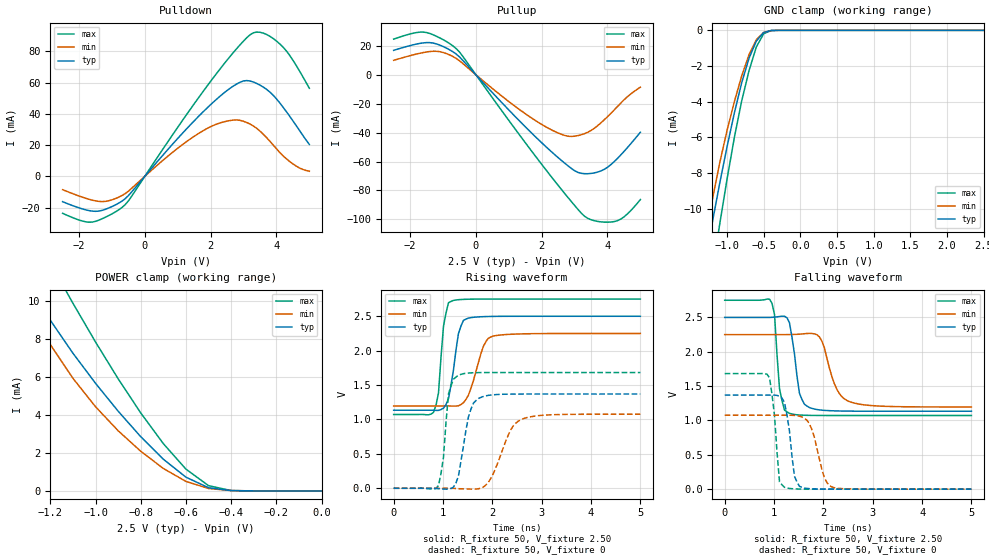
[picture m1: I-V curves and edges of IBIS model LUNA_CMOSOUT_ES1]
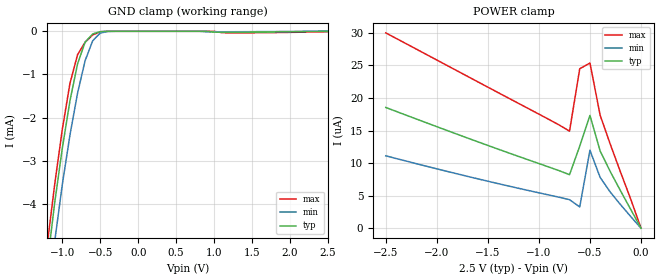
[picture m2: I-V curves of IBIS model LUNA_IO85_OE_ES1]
[IBIS Ver]   3.2
[Comment Char]   |_char
[File name]   sg-9101cx_25v_a.ibs
[File Rev]   1.0
[Date]   2018/09/14 17:35:48
[Source]
[Notes]
[Disclaimer]
This information is for modeling purposes only, and is not guaranteed.
Property of SEIKO EPSON Corp.,
unauthorized reproduction and/or distribution is strictly prohibited.
[Copyright]
Copyright 2018, SEIKO EPSON Corp.
[Component]   SG-9101CA
Si_location Pin
Timing_location Pin
[Manufacturer]   SEIKO EPSON Corp.
| 7050 PKG
| 7050 PKG
[Package]
R_pkg   224m   NA   NA
L_pkg   5.5n   NA   NA
C_pkg   0.144p   NA   NA
[Pin] signal_name   model_name
1   OE   LUNA_IO85_OE_ES1
2   VSS   GND
3   OUT   LUNA_CMOSOUT_ES1
4   VDD   POWER
[Component]   SG-9101CB
Si_location Pin
Timing_location Pin
[Manufacturer]   SEIKO EPSON Corp.
| 5032 PKG
| 5032 PKG
[Package]
R_pkg   200m   NA   NA
L_pkg   2.16n   NA   NA
C_pkg   1.23p   NA   NA
[Pin] signal_name   model_name
1   OE   LUNA_IO85_OE_ES1
2   VSS   GND
3   OUT   LUNA_CMOSOUT_ES1
4   VDD   POWER
[Component]   SG-9101CE
Si_location Pin
Timing_location Pin
[Manufacturer]   SEIKO EPSON Corp.
| 3225 PKG
| 3225 PKG
[Package]
R_pkg   177m   NA   NA
L_pkg   4.5n   NA   NA
C_pkg   0.64p   NA   NA
[Pin] signal_name   model_name
1   OE   LUNA_IO85_OE_ES1
2   VSS   GND
3   OUT   LUNA_CMOSOUT_ES1
4   VDD   POWER
[Component]   SG-9101CG
Si_location Pin
Timing_location Pin
[Manufacturer]   SEIKO EPSON Corp.
| 2520 PKG
| 2520 PKG
[Package]
R_pkg   238m   NA   NA
L_pkg   2.1n   NA   NA
C_pkg   0.38p   NA   NA
[Pin] signal_name   model_name
1   OE   LUNA_IO85_OE_ES1
2   VSS   GND
3   OUT   LUNA_CMOSOUT_ES1
4   VDD   POWER
| Models and submodels in the file (2): LUNA_CMOSOUT_ES1 (3-state), LUNA_IO85_OE_ES1 (Input)
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[Model]   LUNA_CMOSOUT_ES1
Model_type 3-state
Enable Active-High
Polarity Non-Inverting
Vmeas=1.25
C_comp   2.5p   2.0p   3.0p
[Temperature Range] 25   105   -40
[Voltage Range]   2.50   2.25   2.75
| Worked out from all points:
|   slope of the pulldown table from 0 to 0.375 V, typ, clamps not added: 40.3 ohm
|   slope of the pullup table from 0 to 0.375 V, typ, clamps not added: 40.5 ohm
|   GND clamp passes 1 mA (typ) near -0.64 V on its own axis
|   POWER clamp passes 1 mA (typ) near -0.63 V on its own axis
|   falling waveform, R_fixture 50, V_fixture 2.50: 20-80 % time 153ps typ, 284ps min, 106ps max; typ from 2.5 V to 1.13 V
|   falling waveform, R_fixture 50, V_fixture 0: 20-80 % time 142ps typ, 230ps min, 120ps max; typ from 1.37 V to 0 V
|   rising waveform, R_fixture 50, V_fixture 2.50: 20-80 % time 170ps typ, 265ps min, 115ps max; typ from 1.13 V to 2.5 V
|   rising waveform, R_fixture 50, V_fixture 0: 20-80 % time 207ps typ, 362ps min, 123ps max; typ from 0 V to 1.37 V
[Pullup]
-2.5V     16.88mA    9.98mA     24.65mA
-1.5V     22.23mA    15.75mA    29.19mA
-1.1V     20.51mA    15.96mA    25.51mA
-600mV    14.33mA    11.31mA    18.1mA
1.9V      -44.85mA   -32.97mA   -58.98mA
2.7V      -61.14mA   -41.98mA   -82.12mA
3.1V      -67.51mA   -42.09mA   -93.03mA
3.5V      -68.25mA   -38.54mA   -100.3mA
3.9V      -65.45mA   -31.2mA    -101.9mA
4.2V      -60.17mA   -24.44mA   -101.6mA
4.5V      -53.1mA    -17.42mA   -98.33mA
5V        -39.74mA   -8.599mA   -86.32mA
[Pulldown]
-2.5V     -16.25mA   -8.571mA   -23.68mA
-1.6V     -22.29mA   -15.27mA   -29.31mA
-1.1V     -20.31mA   -15.69mA   -25.16mA
-600mV    -14.4mA    -11.1mA    -18.2mA
900mV     21.89mA    16.28mA    28.28mA
1.9V      43.85mA    30.66mA    57.95mA
2.8V      59.13mA    36.05mA    81.88mA
3.3V      60.3mA     32.16mA    91.82mA
3.7V      55.62mA    24.74mA    90.75mA
4.2V      44.25mA    13.13mA    82.67mA
4.6V      32.45mA    6.521mA    70.93mA
5V        20.38mA    3.216mA    56.31mA
[GND Clamp]
-2.5V     -55.19mA   -49.46mA   -64.23mA
-1.3V     -13.11mA   -11.85mA   -16.24mA
-1.2V     -10.77mA   -9.503mA   -13.52mA
-1.1V     -8.591mA   -7.44mA    -10.88mA
-1V       -6.541mA   -5.623mA   -8.358mA
-900mV    -4.635mA   -4.001mA   -6.009mA
-800mV    -2.939mA   -2.563mA   -3.961mA
-700mV    -1.565mA   -1.365mA   -2.263mA
-600mV    -601.2uA   -521.6uA   -925.2uA
-500mV    -121.4uA   -116.4uA   -188.8uA
-300mV    -500.8nA   -1.29uA    -313.5nA
2.5V      140pA      621.1nA    98.8pA
[POWER Clamp]
-2.5V     46.99mA    40.94mA    56.3mA
-1.4V     13.2mA     11.93mA    16.56mA
-1.3V     10.93mA    9.714mA    14.21mA
-1.2V     8.97mA     7.69mA     11.99mA
-1.1V     7.236mA    5.92mA     9.861mA
-1V       5.655mA    4.424mA    7.824mA
-900mV    4.191mA    3.162mA    5.894mA
-700mV    1.665mA    1.179mA    2.483mA
-600mV    721.7uA    498.7uA    1.143mA
-500mV    167.2uA    126.9uA    275.1uA
-400mV    16.41uA    18.75uA    19.76uA
0V        140pA      780.7pA    121.2pA
[Falling Waveform]
R_fixture=50
V_fixture=2.50
V_fixture_min=2.25
V_fixture_max=2.75
0s        2.5V       2.25V      2.75V
959.6ps   2.502V     2.25V      2.704V
1.01ns    2.504V     2.25V      2.539V
1.111ns   2.513V     2.25V      1.46V
1.313ns   2.422V     2.251V     1.103V
1.515ns   1.395V     2.256V     1.079V
1.717ns   1.188V     2.268V     1.074V
1.97ns    1.15V      2.156V     1.073V
2.525ns   1.136V     1.275V     1.072V
5ns       1.134V     1.196V     1.072V
[Falling Waveform]
R_fixture=50
V_fixture=0
V_fixture_min=0
V_fixture_max=0
0s        1.37V      1.076V     1.682V
909.1ps   1.37V      1.076V     1.62V
1.01ns    1.369V     1.076V     1.067V
1.111ns   1.354V     1.076V     106.5mV
1.212ns   1.26V      1.076V     26.99mV
1.414ns   188mV      1.074V     4.222mV
1.515ns   41.08mV    1.063V     1.872mV
1.717ns   7.173mV    952.4mV    388uV
2.172ns   507.1uV    33.38mV    22.45uV
5ns       0V         1.7uV      0V
[Rising Waveform]
R_fixture=50
V_fixture=2.50
V_fixture_min=2.25
V_fixture_max=2.75
0s        1.134V     1.196V     1.072V
808.1ps   1.134V     1.196V     1.104V
909.1ps   1.132V     1.196V     1.386V
1.01ns    1.164V     1.196V     2.356V
1.162ns   1.499V     1.195V     2.715V
1.313ns   2.248V     1.199V     2.741V
1.515ns   2.474V     1.353V     2.748V
1.818ns   2.494V     2.062V     2.75V
2.02ns    2.498V     2.213V     2.75V
5ns       2.5V       2.25V      2.75V
[Rising Waveform]
R_fixture=50
V_fixture=0
V_fixture_min=0
V_fixture_max=0
0s        0V         0V         0V
909.1ps   -5.742mV   -9.93uV    39.89mV
1.01ns    -11.2mV    84.96uV    453.7mV
1.111ns   -12.61mV   333.4uV    1.371V
1.313ns   177.7mV    -6.019mV   1.643V
1.515ns   1.035V     -11.08mV   1.675V
1.768ns   1.321V     2.604mV    1.681V
1.97ns    1.355V     144.3mV    1.682V
2.576ns   1.37V      995.6mV    1.682V
5ns       1.37V      1.076V     1.682V
[Ramp]
R_load=50
dV/dt_r   8.220E-1/2.067E-10   6.457E-1/3.597E-10   1.009E+0/1.052E-10
dV/dt_f   8.193E-1/1.483E-10   6.322E-1/2.787E-10   1.007E+0/1.056E-10
|[End   LUNA_CMOSOUT_ES1
[Model]   LUNA_IO85_OE_ES1
Model_type Input
Enable Active-Low
Polarity Non-Inverting
Vinh=1.93
Vinl=0.67
C_comp   2.5p   2.0p   3.0p
[Temperature Range] 25   105   -40
[Voltage Range]   2.50   2.25   2.75
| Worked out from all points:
|   GND clamp passes 1 mA (typ) near -0.83 V on its own axis
[GND Clamp]
-2.5V     -32.2mA    -31.31mA   -34.3mA
-1.2V     -5.408mA   -6.351mA   -4.953mA
-1.1V     -3.959mA   -4.854mA   -3.533mA
-1V       -2.702mA   -3.543mA   -2.264mA
-900mV    -1.611mA   -2.406mA   -1.207mA
-800mV    -755.7uA   -1.435mA   -544uA
-700mV    -251.7uA   -679.9uA   -254uA
-600mV    -60.42uA   -218.4uA   -84.78uA
-500mV    -8.306uA   -39.73uA   -10.67uA
-400mV    -801.3nA   -4.121uA   -821nA
1.2V      -21.43uA   -11.22uA   -36.93uA
2.5V      102pA      4.547uA    -9.898uA
[POWER Clamp]
-2.5V     18.55uA    11.12uA    30.01uA
-1.6V     13.28uA    7.586uA    22.5uA
-900mV    9.38uA     5.089uA    16.69uA
-700mV    8.214uA    4.376uA    14.9uA
-600mV    12.61uA    3.264uA    24.49uA
-500mV    17.33uA    11.98uA    25.38uA
-400mV    11.86uA    7.796uA    17.35uA
-300mV    8.666uA    5.523uA    12.86uA
-100mV    2.864uA    1.778uA    4.438uA
0V        101.8pA    233pA      102.9pA
